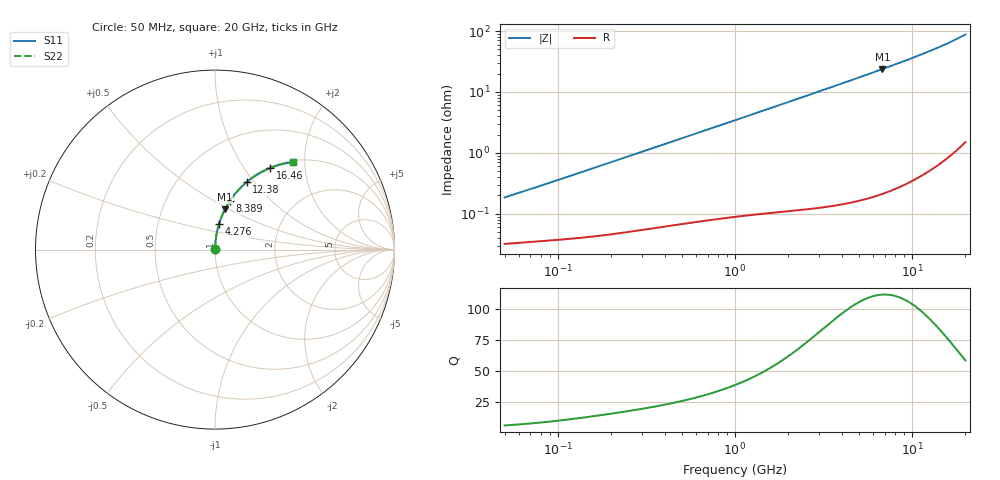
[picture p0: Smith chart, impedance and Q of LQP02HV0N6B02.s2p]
!Murata Part Number: LQP02HV0N6B02
!These Parameters are Measured in Series Mode Connection
!  o--[Z]--o
!Port1  Port2
!  o-------o
!Freq. Start=50[MHz] Stop=20[GHz], 401[Steps]
# Hz S RI R 50
!Freq.(Hz) S11(Real) S11(Imag) S21(Real) S21(Imag) S12(Real) S12(Imag) S22(Real) S22(Imag)
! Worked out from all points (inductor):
!   401 points, 50 MHz to 20 GHz, reference 50 ohm
!   read as one part in series: L = 576 pH near 51.52 MHz
!   highest Q = 112 at 6.802 GHz (marker M1), where L = 555 pH
!   S11 on the Smith chart (normalised r, x): 50 MHz: 1.00, +0.00; 4.276 GHz: 1.00, +0.29; 8.389 GHz: 1.01, +0.59; 12.38 GHz: 1.01, +0.92; 16.46 GHz: 1.02, +1.32; 20 GHz: 1.03, +1.75
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5e7  0.000324 0.00183  0.9997 -0.00183  0.9997 -0.00183  0.000324 0.00183
5.152053e7  0.000326 0.00188  0.9997 -0.00188  0.9997 -0.00188  0.000326 0.00188
6.746414e7  0.000349 0.00244  0.9997 -0.00244  0.9997 -0.00244  0.000349 0.00244
1.364002e8  0.000429 0.00484  0.9996 -0.00484  0.9996 -0.00484  0.000429 0.00484
3.721004e8  0.000765 0.0129  0.9992 -0.0129  0.9992 -0.0129  0.000765 0.0129
6.380365e8  0.00123 0.022  0.9988 -0.022  0.9988 -0.022  0.00123 0.022
1e9  0.00206 0.0342  0.9979 -0.0342  0.9979 -0.0342  0.00206 0.0342
1.714689e9  0.00446 0.0582  0.9955 -0.0582  0.9955 -0.0582  0.00446 0.0582
2.728004e9  0.00979 0.0922  0.9902 -0.0922  0.9902 -0.0922  0.00979 0.0922
3.415248e9  0.0147 0.115  0.9853 -0.115  0.9853 -0.115  0.0147 0.115
4.275624e9  0.0225 0.1433  0.9775 -0.1433  0.9775 -0.1433  0.0225 0.1433
5.433528e9  0.0356 0.1807  0.9644 -0.1807  0.9644 -0.1807  0.0356 0.1807
6.802353e9  0.0551 0.2237  0.9449 -0.2237  0.9449 -0.2237  0.0551 0.2237
7.442007e9  0.0656 0.2432  0.9344 -0.2432  0.9344 -0.2432  0.0656 0.2432
8.389408e9  0.083 0.2714  0.917 -0.2714  0.917 -0.2714  0.083 0.2714
1.034674e10  0.1251 0.326  0.8749 -0.326  0.8749 -0.326  0.1251 0.326
1.238412e10  0.1776 0.3768  0.8224 -0.3768  0.8224 -0.3768  0.1776 0.3768
1.438523e10  0.237 0.4193  0.763 -0.4193  0.763 -0.4193  0.237 0.4193
1.646126e10  0.3059 0.454  0.6941 -0.454  0.6941 -0.454  0.3059 0.454
1.828096e10  0.3713 0.4756  0.6287 -0.4756  0.6287 -0.4756  0.3713 0.4756
1.940974e10  0.4136 0.4843  0.5864 -0.4843  0.5864 -0.4843  0.4136 0.4843
2e10  0.4361 0.4874  0.5639 -0.4874  0.5639 -0.4874  0.4361 0.4874
